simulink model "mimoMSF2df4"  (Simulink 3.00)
settings: Solver=ode45  StartTime=0.0  StopTime=50.0  RelTol=1e-3
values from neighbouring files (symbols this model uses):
  Disturb = Setpoint    [mimo_MSF1DF_sim.m]    (also in mimo_MSF2DF_sim.m)
  K = 1/kpd    [imc2pseucon.m]    (also in imc2pseudo.m)
  Satlb = temp1    [cback.m]    (also in imcmenu.m = str2num(satlbs))
  Satub = temp1    [cback.m]    (also in imcmenu.m = str2num(satubs))
  Setpoint = zeros(1,n)    [mimo_MSF1DF_sim.m]    (also in mimo_MSF2DF_sim.m)
undefined symbols (not defined in the file or in its folder): Ds, input_delay, Kdelay, Ksp, T
libraries: MIMO_lib x20, simulink3 x19

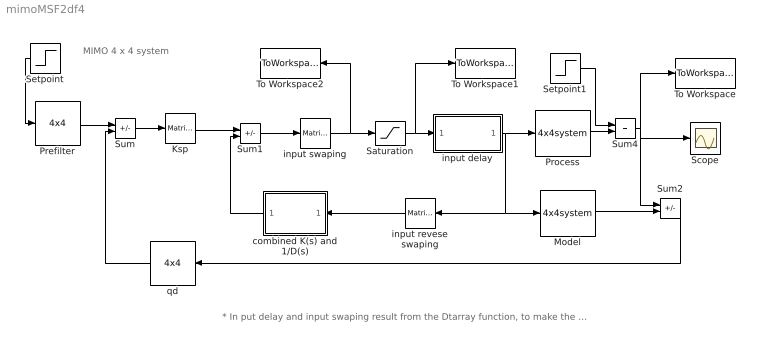
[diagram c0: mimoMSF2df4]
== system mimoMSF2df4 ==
  note: * In put delay and input swaping result from the Dtarray function, to make the system be able to be decoupled.
  note: MIMO 4 x 4 system
  Ksp : simulink3/Math/Matrix Gain  K=Ksp
  Model : MIMO_lib/4x4system  num=Mnum  den=Mden  dead=Mdead
  Prefilter : MIMO_lib/4x4  num=prefilnum  den=prefilden
  Process : MIMO_lib/4x4system  num=Pnum  den=Pden  dead=Pdead
  Saturation : Saturate  UpperLimit=Satub  LowerLimit=Satlb
  Scope : Scope
  Setpoint : Step  Orientation=left  Time=0  Before=0  After=[Setpoint]  SampleTime=0
  Setpoint1 : Step  Time=0  Before=0  After=[Disturb]  SampleTime=0
  Sum : Sum  Inputs=+-  SaturateOnIntegerOverflow=on
  Sum1 : Sum  Inputs=+-  SaturateOnIntegerOverflow=on
  Sum2 : Sum  Inputs=+-  SaturateOnIntegerOverflow=on
  Sum4 : Sum  Inputs=++  SaturateOnIntegerOverflow=on
  To Workspace : ToWorkspace  VariableName=yout  SampleTime=0  SaveFormat=Matrix
  To Workspace1 : ToWorkspace  VariableName=sat_effort  SampleTime=0  SaveFormat=Matrix
  To Workspace2 : ToWorkspace  VariableName=unsat_effort  SampleTime=0  SaveFormat=Matrix
  combined K(s) and 1/D(s) : Subsystem  Orientation=left  mask(ksds){Ksp=Ksp, Ds=Ds, Kdelay=Kdelay, K=K}
      mask prompts: Ds "D(s)"; Kdelay "Bdelay"; K "B*(s)"
  input delay : Subsystem  mask(input delay){input_delay=input_delay}
      mask prompts: input_delay "Input Delay (vector)"
  input revese swaping : simulink3/Math/Matrix Gain  Orientation=left  K=T
  input swaping : simulink3/Math/Matrix Gain  K=inv(T)
  qd : MIMO_lib/4x4  Orientation=left  num=qdnum  den=qdden
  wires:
  Ksp/1 -> Sum1/1
  combined K(s) and 1/D(s)/1(Out1) -> Sum1/2
  Sum/1 -> Ksp/1
  input revese swaping/1 -> combined K(s) and 1/D(s)/1(In1)
  Model/1 -> Sum2/2
  Process/1 -> Sum4/2
  Setpoint1/1 -> Sum4/1
  Sum4/1 -> Sum2/1, To Workspace/1, Scope/1
  input swaping/1 -> Saturation/1, To Workspace2/1
  Sum1/1 -> input swaping/1
  input delay/1(Out1) -> Process/1, Model/1, input revese swaping/1
  Saturation/1 -> input delay/1(In1), To Workspace1/1
  Prefilter/1 -> Sum/1
  Setpoint/1 -> Prefilter/1
  qd/1 -> Sum/2
  Sum2/1 -> qd/1

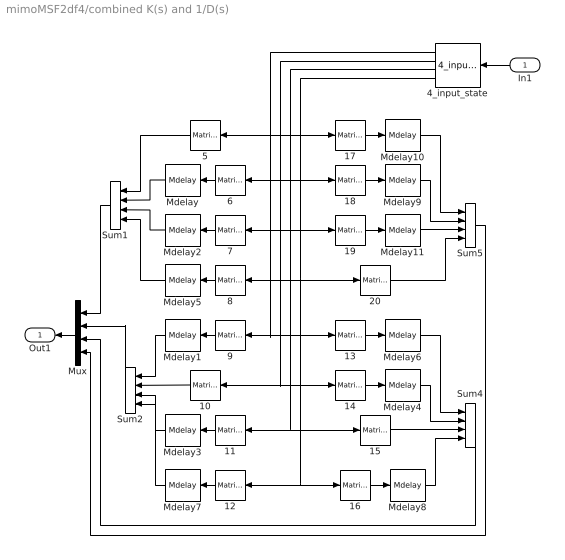
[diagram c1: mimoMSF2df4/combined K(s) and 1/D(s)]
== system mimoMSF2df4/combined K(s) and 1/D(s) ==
  In1 : Inport  Orientation=left  Port=1  PortWidth=-1  SampleTime=-1  DataType=auto
  10 : simulink3/Math/Matrix Gain  Orientation=left  K="[zeros(1,length(Ds{2})-length(K{2,2}))  K{2,2}]"
  11 : simulink3/Math/Matrix Gain  Orientation=left  K="[zeros(1,length(Ds{3})-length(K{2,3}))  K{2,3}]"
  12 : simulink3/Math/Matrix Gain  Orientation=left  K="[zeros(1,length(Ds{4})-length(K{2,4}))  K{2,4}]"
  13 : simulink3/Math/Matrix Gain  K="[zeros(1,length(Ds{1})-length(K{3,1}))  K{3,1}]"
  14 : simulink3/Math/Matrix Gain  K="[zeros(1,length(Ds{2})-length(K{3,2}))  K{3,2}]"
  15 : simulink3/Math/Matrix Gain  K="[zeros(1,length(Ds{3})-length(K{3,3}))  K{3,3}]"
  16 : simulink3/Math/Matrix Gain  K="[zeros(1,length(Ds{4})-length(K{3,4}))  K{3,4}]"
  17 : simulink3/Math/Matrix Gain  K="[zeros(1,length(Ds{1})-length(K{4,1}))  K{4,1}]"
  18 : simulink3/Math/Matrix Gain  K="[zeros(1,length(Ds{2})-length(K{4,2}))  K{4,2}]"
  19 : simulink3/Math/Matrix Gain  K="[zeros(1,length(Ds{3})-length(K{4,3}))  K{4,3}]"
  20 : simulink3/Math/Matrix Gain  K="[zeros(1,length(Ds{4})-length(K{4,4}))  K{4,4}]"
  4_input_state : MIMO_lib/4_input_state  Orientation=left  Ds=Ds
  5 : simulink3/Math/Matrix Gain  Orientation=left  K="[zeros(1,length(Ds{1})-length(K{1,1}))  K{1,1}]"
  6 : simulink3/Math/Matrix Gain  Orientation=left  K=[zeros(1,length(Ds{2})-length(K{1,2})) K{1,2}]
  7 : simulink3/Math/Matrix Gain  Orientation=left  K="[zeros(1,length(Ds{3})-length(K{1,3}))  K{1,3}]"
  8 : simulink3/Math/Matrix Gain  Orientation=left  K="[zeros(1,length(Ds{4})-length(K{1,4}))  K{1,4}]"
  9 : simulink3/Math/Matrix Gain  Orientation=left  K="[zeros(1,length(Ds{1})-length(K{2,1}))  K{2,1}]"
  Mdelay : MIMO_lib/Mdelay  Orientation=left  Mdelay=Kdelay(1,2)
  Mdelay1 : MIMO_lib/Mdelay  Orientation=left  Mdelay=Kdelay(2,1)
  Mdelay10 : MIMO_lib/Mdelay  Mdelay=Kdelay(4,1)
  Mdelay11 : MIMO_lib/Mdelay  Mdelay=Kdelay(4,3)
  Mdelay2 : MIMO_lib/Mdelay  Orientation=left  Mdelay=Kdelay(1,3)
  Mdelay3 : MIMO_lib/Mdelay  Orientation=left  Mdelay=Kdelay(2,3)
  Mdelay4 : MIMO_lib/Mdelay  Mdelay=Kdelay(3,2)
  Mdelay5 : MIMO_lib/Mdelay  Orientation=left  Mdelay=Kdelay(1,4)
  Mdelay6 : MIMO_lib/Mdelay  Mdelay=Kdelay(3,1)
  Mdelay7 : MIMO_lib/Mdelay  Orientation=left  Mdelay=Kdelay(2,4)
  Mdelay8 : MIMO_lib/Mdelay  Mdelay=Kdelay(3,4)
  Mdelay9 : MIMO_lib/Mdelay  Mdelay=Kdelay(4,2)
  Mux : Mux  Orientation=left  Inputs=4
  Sum1 : Sum  Orientation=left  Inputs=++++  SaturateOnIntegerOverflow=on
  Sum2 : Sum  Orientation=left  Inputs=++++  SaturateOnIntegerOverflow=on
  Sum4 : Sum  Inputs=++++  SaturateOnIntegerOverflow=on
  Sum5 : Sum  Inputs=++++  SaturateOnIntegerOverflow=on
  Out1 : Outport  Orientation=left  Port=1
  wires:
  Sum2/1 -> Mux/2
  Mux/1 -> Out1/1
  Sum1/1 -> Mux/1
  9/1 -> Mdelay1/1
  Mdelay1/1 -> Sum2/1
  10/1 -> Sum2/2
  11/1 -> Mdelay3/1
  Mdelay3/1 -> Sum2/3
  In1/1 -> 4_input_state/1
  5/1 -> Sum1/1
  Mdelay/1 -> Sum1/2
  Mdelay2/1 -> Sum1/3
  6/1 -> Mdelay/1
  7/1 -> Mdelay2/1
  8/1 -> Mdelay5/1
  Mdelay5/1 -> Sum1/4
  12/1 -> Mdelay7/1
  Mdelay7/1 -> Sum2/4
  Mdelay6/1 -> Sum4/1
  15/1 -> Sum4/3
  Sum4/1 -> Mux/3
  13/1 -> Mdelay6/1
  14/1 -> Mdelay4/1
  16/1 -> Mdelay8/1
  Mdelay8/1 -> Sum4/4
  Mdelay4/1 -> Sum4/2
  Mdelay10/1 -> Sum5/1
  17/1 -> Mdelay10/1
  18/1 -> Mdelay9/1
  Mdelay9/1 -> Sum5/2
  19/1 -> Mdelay11/1
  Mdelay11/1 -> Sum5/3
  20/1 -> Sum5/4
  Sum5/1 -> Mux/4
  4_input_state/4 -> 8/1, 12/1, 16/1, 20/1
  4_input_state/3 -> 7/1, 11/1, 15/1, 19/1
  4_input_state/2 -> 6/1, 10/1, 14/1, 18/1
  4_input_state/1 -> 5/1, 9/1, 13/1, 17/1

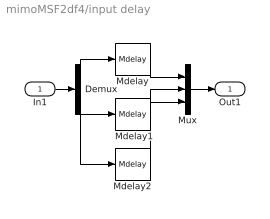
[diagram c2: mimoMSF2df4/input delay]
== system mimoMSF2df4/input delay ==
  In1 : Inport  Port=1  PortWidth=-1  SampleTime=-1  DataType=auto
  Demux : Demux  Outputs=3
  Mdelay : MIMO_lib/Mdelay  Mdelay=input_delay(1)
  Mdelay1 : MIMO_lib/Mdelay  Mdelay=input_delay(2)
  Mdelay2 : MIMO_lib/Mdelay  Mdelay=input_delay(3)
  Mux : Mux  Inputs=3
  Out1 : Outport  Port=1
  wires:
  Mux/1 -> Out1/1
  In1/1 -> Demux/1
  Demux/1 -> Mdelay/1
  Demux/2 -> Mdelay1/1
  Mdelay/1 -> Mux/1
  Mdelay1/1 -> Mux/2
  Demux/3 -> Mdelay2/1
  Mdelay2/1 -> Mux/3
